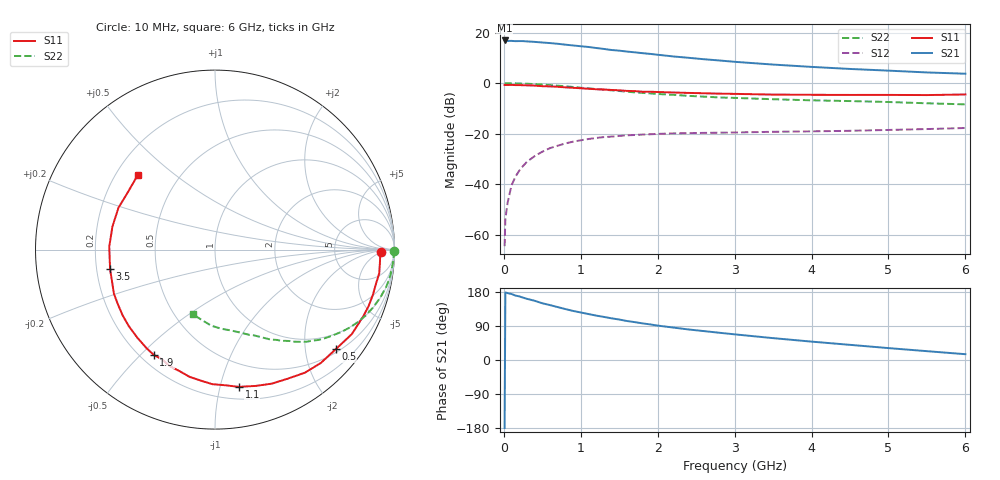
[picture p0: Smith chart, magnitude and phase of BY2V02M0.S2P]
! SIEMENS Small Signal Semiconductors
! BFY420
! Si NPN RF SIEGET Grounded Emitter Transistor in MICRO-X
! VCE = 2 V  IC = 2 mA
! Common Emitter S-Parameters:  October  1996
# GHz  S  MA  R  50
!  f  S11  S21  S12  S22
! GHz  MAG  ANG  MAG  ANG  MAG  ANG  MAG  ANG
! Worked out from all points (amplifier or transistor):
!   36 points, 10 MHz to 6 GHz, reference 50 ohm
!   highest |S21| = 16.9 dB at 10 MHz (marker M1)
!   |S21| within 3 dB of that: start of sweep to 1.204 GHz
!   unconditionally stable (mu >= 1): 3.995 GHz to end of sweep
!   at 250 MHz: K = 0.06, MSG = 24.7 dB, |S12| = -32.7 dB
!   at 1.4 GHz: K = 0.29, MSG = 17.1 dB, |S12| = -21.1 dB
!   at 6 GHz: K = 1.24, MAG = 7.8 dB, |S12| = -17.7 dB
!   S11 on the Smith chart (normalised r, x): 10 MHz: 24, -4; 500 MHz: 0.58, -2.68; 1.1 GHz: 0.30, -1.15; 1.9 GHz: 0.25, -0.55; 3.5 GHz: 0.26, -0.09; 6 GHz: 0.29, +0.37
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0.01  0.9231 -0.8  6.99 -179.5  0.0006 110.3  0.9974 -0.4
0.02  0.9208 -1.8  6.928 178.4  0.0021 81.9  0.9988 -0.8
0.05  0.9216 -4.1  6.829 176.4  0.0044 86.9  0.9963 -2.0
0.1  0.9246 -8.2  6.856 174.2  0.0096 85.2  0.9939 -4.2
0.15  0.9168 -12.0  6.773 170.1  0.0141 83.2  0.9905 -6.3
0.2  0.915 -16.1  6.795 167.9  0.0186 81.5  0.9877 -8.2
0.25  0.9117 -20.2  6.785 164.5  0.0231 77.4  0.9821 -10.3
0.4  0.896 -31.7  6.553 156.3  0.0361 71.9  0.9588 -16.2
0.5  0.8721 -39.5  6.363 149.7  0.0442 67.5  0.9389 -19.9
0.7  0.8495 -53.8  6.011 139.6  0.0581 59.7  0.8926 -26.9
0.8  0.8258 -60.5  5.772 134.4  0.0644 55.3  0.8669 -30.1
0.9  0.811 -67.1  5.568 129.5  0.0699 51.9  0.8418 -32.9
1.1  0.7762 -80.1  5.198 121.3  0.0788 46.0  0.79 -38.5
1.4  0.7343 -96.2  4.529 110.0  0.0879 38.5  0.7224 -45.3
1.6  0.7041 -106.7  4.214 102.9  0.0932 34.3  0.6792 -49.1
1.9  0.6787 -120.2  3.796 94.0  0.0977 29.2  0.6277 -54.1
2.2  0.6545 -131.4  3.379 85.7  0.1018 25.1  0.5891 -58.3
2.8  0.621 -150.5  2.813 71.9  0.1051 19.6  0.5224 -65.9
3.5  0.5946 -169.5  2.334 57.7  0.1094 15.8  0.4816 -73.4
4.5  0.5857 167.4  1.911 40.0  0.1145 12.7  0.443 -85.2
5.5  0.5819 145.7  1.63 23.3  0.1239 10.9  0.4003 -100.1
6  0.5982 136.0  1.539 15.3  0.1301 10.1  0.3815 -108.8
